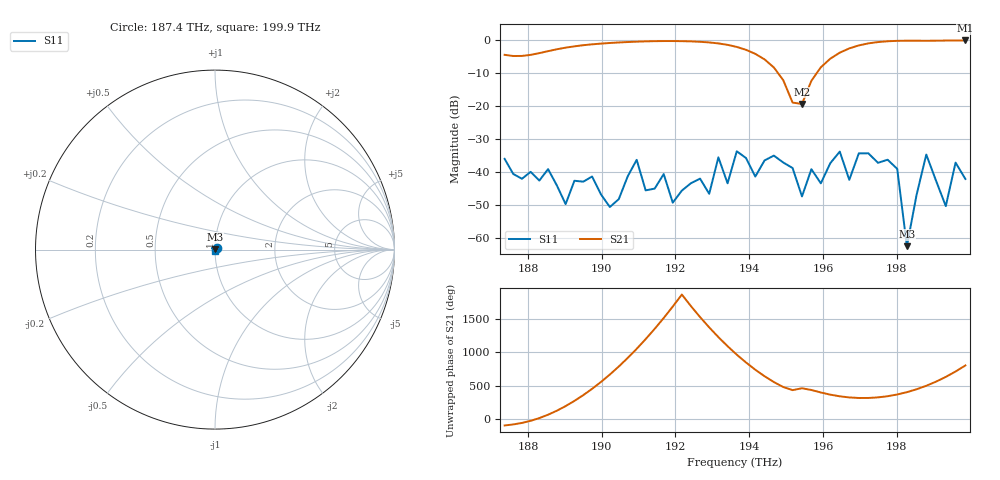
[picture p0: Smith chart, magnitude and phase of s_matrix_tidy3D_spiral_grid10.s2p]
[Version] 2.0
# Hz S RI
[Number of Ports] 2
[Two-Port Data Order] 12_21
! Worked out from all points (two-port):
!   51 points, 187.4 THz to 199.9 THz, reference 50 ohm
!   highest |S21| = -0.06 dB at 199.9 THz (marker M1); lowest = -19.3 dB at 195.4 THz (marker M2)
!   |S21| within 3 dB of the highest: 188.6 THz to 193.9 THz (5.297 THz wide, 2.77 % of centre); 196.6 THz to end of sweep
!   lowest |S11| = -62.5 dB at 198.3 THz (marker M3), VSWR 1.00, Z = 50 + j0.0658 ohm
!   |S11| at or under -10 dB: start of sweep to end of sweep
!   S12 and S22 are empty: the file has one direction only
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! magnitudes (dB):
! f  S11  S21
! 187.4 THz  -36.0  -4.4
! 189 THz  -49.7  -2.2
! 189.5 THz  -42.9  -1.5
! 190.2 THz  -50.6  -0.8
! 191 THz  -36.3  -0.4
! 191.2 THz  -45.6  -0.3
! 191.7 THz  -40.6  -0.2
! 191.9 THz  -49.3  -0.2
! 192.9 THz  -46.6  -0.7
! 193.2 THz  -35.5  -1.0
! 193.7 THz  -33.7  -2.0
! 195.4 THz  -47.4  -19.3
! 195.9 THz  -43.4  -8.2
! 196.5 THz  -33.8  -3.8
! 196.7 THz  -42.4  -2.5
! 197 THz  -34.3  -1.6
! 198 THz  -39.0  -0.2
! 198.3 THz  -62.5  -0.1
! 198.8 THz  -34.7  -0.2
! 199.3 THz  -50.3  -0.1
! 199.6 THz  -37.1  -0.1
! 199.9 THz  -42.1  -0.1
